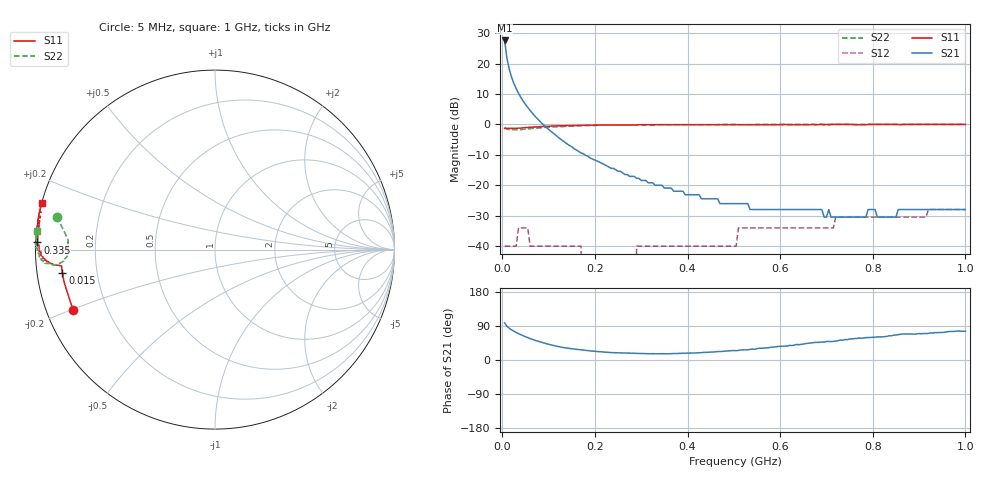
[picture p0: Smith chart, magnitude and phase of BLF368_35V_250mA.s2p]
! Filename:  BLF368_35V_250mA.s2p
! Philips part #: BLF368  !date: 21-05-2003
!35V @250 mA
!D:\Vee measurements\measurement data\VDMOST\BLF368\35V_250mA_#1
# HZ S MA R 50
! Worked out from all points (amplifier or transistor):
!   200 points, 5 MHz to 1 GHz, reference 50 ohm
!   highest |S21| = 27.6 dB at 5 MHz (marker M1)
!   |S21| within 3 dB of that: start of sweep to 7.56 MHz
!   S11 on the Smith chart (normalised r, x): 5 MHz: 0.08, -0.20; 15 MHz: 0.08, -0.08; 335 MHz: 0.01, +0.02; 1 GHz: -0.00, +0.13
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5000000  0.86 -156.9  23.97 98.1  0.01 -3.2  0.9 168.3
1e7  0.86 -167.8  12.21 89.2  0.01 20.7  0.84 173.8
1.5e7  0.86 -171.3  8.1 83.8  0.01 22.3  0.82 176.3
2e7  0.86 -172.9  5.98 79.6  0.01 18.7  0.82 178.1
2.5e7  0.86 -173.5  4.72 76.1  0.01 13.9  0.82 179.4
3e7  0.86 -173.9  3.88 72.7  0.01 8.9  0.82 -179.7
3.5e7  0.87 -174.1  3.26 69.5  0.02 4.5  0.82 -178.8
5e7  0.89 -174.4  2.13 61.4  0.02 -6.4  0.84 -176.4
5.5e7  0.89 -174.5  1.9 58.9  0.02 -9.4  0.84 -175.9
6e7  0.9 -174.6  1.7 56.5  0.01 -12.2  0.85 -175.5
9e7  0.93 -175.5  0.97 44.9  0.01 -23.7  0.89 -174.5
1.7e8  0.97 -178.2  0.34 26.7  0.01 -22.4  0.95 -175.6
1.75e8  0.97 -178.3  0.33 26.1  0 -20.4  0.96 -175.7
2.85e8  0.98 178.8  0.14 17.7  0 66.8  0.98 -178.0
2.9e8  0.98 178.6  0.13 17.3  0.01 68.6  0.98 -178.1
3.35e8  0.99 177.7  0.1 16.5  0.01 76.7  0.98 -178.8
3.4e8  0.99 177.5  0.1 16.4  0.01 76.9  0.99 -178.8
5.05e8  0.99 174.3  0.05 24.5  0.01 88.5  1 179.0
5.1e8  0.99 174.2  0.05 25.3  0.02 88.6  0.99 179.0
6.7e8  1 171.3  0.04 45.6  0.02 90.8  1 177.2
8.35e8  1 168.3  0.03 63.8  0.03 93.4  1 175.7
1e9  1 165.1  0.04 75.8  0.04 92.6  1 173.9
